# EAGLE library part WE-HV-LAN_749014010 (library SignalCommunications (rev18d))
WE-LAN HV LAN-Transformer Characteristics: •Compliant with IEEE802.3 and 802.3af standards •Operating temperature: 0 °C to +70 °C •SMD •4 kV Hipot test Applications: •Ethernet •Compliant with most IC's for Ethernet applications like Intel, AMD, Conexant, Realtek, etc. •Hub, Router, Switches, medical applications Details see: http://katalog.we-online.de/en/pbs/WE-LAN/749014010? Updated by Dan Xu 2014-07-08 2014 (C) Würth Elektronik
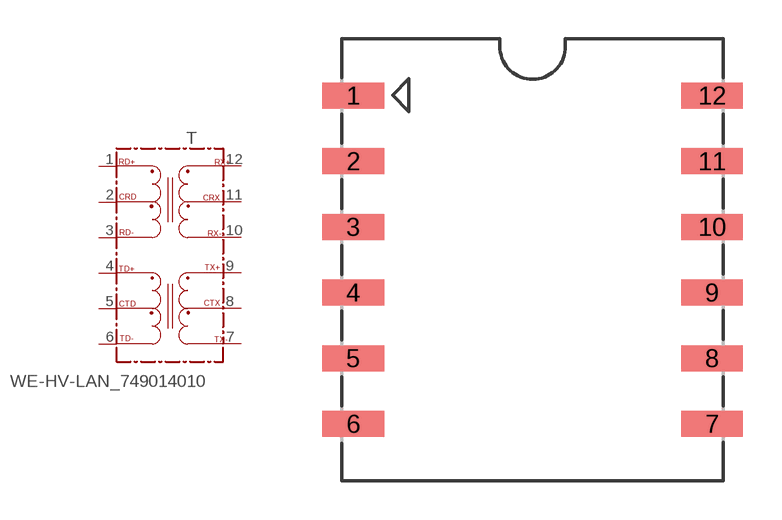
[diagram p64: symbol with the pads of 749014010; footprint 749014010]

Designator prefix T

## WE-HV-LAN_749014010  [749014010]
1  RD+
2  CRD
3  RD-
4  TD+
5  CTD
6  TD-
7  TX-
8  CTX
9  TX+
10  RX-
11  CRX
12  RX+

## Footprint 749014010 (pad centres in mm)
MAX Height=8.40 mm
smd 2.39 x 1: 1 -6.935,6.35; 2 -6.935,3.81; 3 -6.935,1.27; 4 -6.935,-1.27; 5 -6.935,-3.81; 6 -6.935,-6.35; 7 6.935,-6.35; 8 6.935,-3.81; 9 6.935,-1.27; 10 6.935,1.27; 11 6.935,3.81; 12 6.935,6.35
